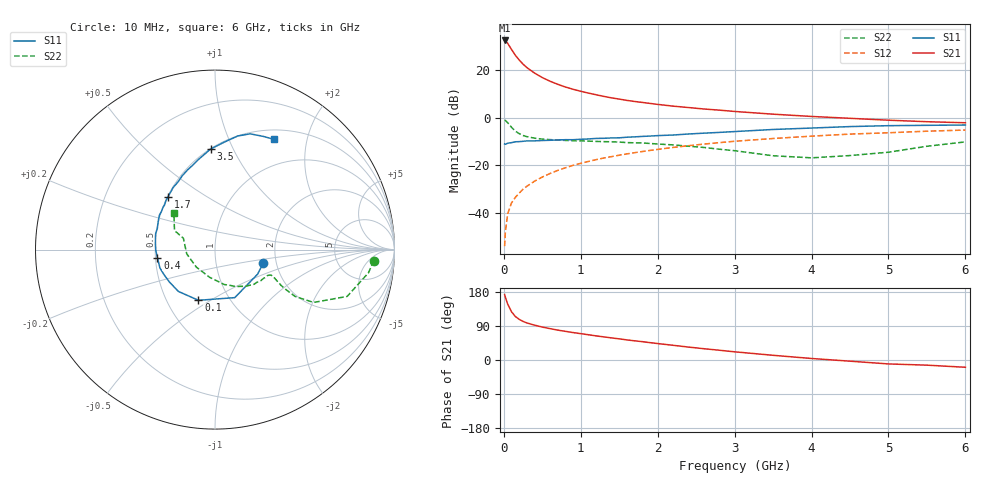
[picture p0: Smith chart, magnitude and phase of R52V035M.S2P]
! SIEMENS Small Signal Semiconductors
! BFR183
! Si NPN RF Bipolar Junction Transistor in SOT23
! VCE = 2 V  IC = 35 mA
! Common Emitter S-Parameters:  May  1996
# GHz  S  MA  R  50
!  f  S11  S21  S12  S22
! GHz  MAG  ANG  MAG  ANG  MAG  ANG  MAG  ANG
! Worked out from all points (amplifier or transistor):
!   36 points, 10 MHz to 6 GHz, reference 50 ohm
!   highest |S21| = 32.3 dB at 10 MHz (marker M1)
!   |S21| within 3 dB of that: start of sweep to 84.75 MHz
!   unconditionally stable (mu >= 1): start of sweep to 12.87 MHz; 287.5 MHz to 2.578 GHz
!   at 250 MHz: K = 0.97, MSG = 26.2 dB, |S12| = -30.1 dB
!   at 1.4 GHz: K = 1.08, MAG = 10.6 dB, |S12| = -16.4 dB
!   at 6 GHz: K = 0.94, MSG = 1.5 dB, |S12| = -5.3 dB
!   S11 on the Smith chart (normalised r, x): 10 MHz: 1.71, -0.28; 100 MHz: 0.72, -0.44; 400 MHz: 0.51, -0.05; 1.7 GHz: 0.50, +0.35; 3.5 GHz: 0.50, +0.82; 6 GHz: 0.62, +1.49
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0.01  0.2792 -15.5  41.36 172.7  0.002 83.9  0.8872 -4.0
0.02  0.274 -29.9  40.58 165.6  0.004 80.6  0.8647 -8.6
0.05  0.2894 -67.6  35.99 147.6  0.0095 71.5  0.7811 -19.5
0.1  0.2972 -108.1  26.74 127.2  0.0162 69.6  0.6232 -28.2
0.15  0.3097 -131.2  20.19 114.7  0.0211 69.7  0.5178 -30.3
0.2  0.3118 -144.9  16.06 107.3  0.026 70.4  0.4589 -29.5
0.25  0.317 -154.5  13.15 101.8  0.0314 71.5  0.4201 -28.5
0.3  0.3235 -161.6  11.13 97.7  0.0362 72.5  0.3962 -27.3
0.4  0.3238 -172.1  8.539 91.9  0.0462 73.6  0.3684 -25.6
0.5  0.3296 -178.9  6.883 86.9  0.0564 74.3  0.3524 -24.7
0.6  0.3332 174.6  5.774 82.8  0.0668 74.0  0.3437 -24.5
0.7  0.3379 169.1  4.979 78.9  0.0776 73.9  0.3369 -25.0
0.9  0.3422 159.9  3.914 72.4  0.0993 72.2  0.3262 -26.3
1.1  0.3552 152.5  3.253 66.6  0.1198 70.6  0.3198 -29.2
1.4  0.373 141.1  2.585 58.3  0.1514 67.7  0.3097 -33.6
1.7  0.3926 131.9  2.17 50.6  0.1829 64.2  0.2942 -38.9
2.2  0.4295 118.7  1.733 38.8  0.2356 58.1  0.2665 -50.2
3  0.5073 101.0  1.34 21.6  0.3175 47.3  0.2013 -75.1
3.5  0.5611 92.5  1.175 12.4  0.3629 40.1  0.1576 -100.6
4.5  0.6454 78.7  0.962 -3.1  0.4491 26.4  0.1592 -171.4
5.5  0.6857 66.9  0.817 -13.6  0.5164 14.2  0.2494 154.8
6  0.6967 61.8  0.776 -19.2  0.5461 6.5  0.3079 138.1
